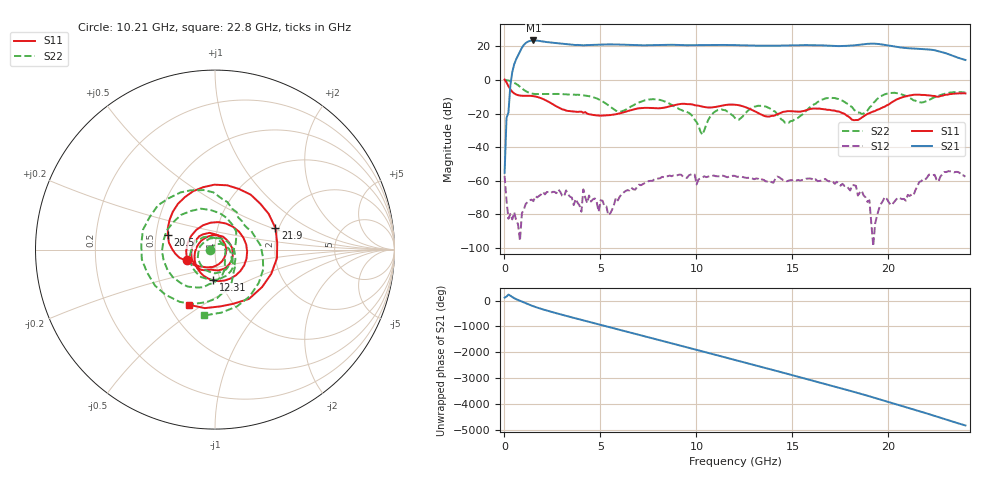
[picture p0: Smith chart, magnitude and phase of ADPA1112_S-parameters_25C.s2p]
! Analog Devices Inc.
! Device:  ADPA1112
! Description: 15 W, GaN Power Amplifier
! Frequency:  1 GHz to 22 GHz
! Package:
! Conditions:	Vdd = 28.0 V
!		Idd = 600 mA
!		Temp = +25 C
! The board loss has been subtracted from S21 Magnitude. Reference for all other parameters are at the connectors.
! Misc:JB
! Note: Analog Devices supplies this data as a sample of measured data for this product.
! Your particular data for this product may vary.
! Analog Devices reserves the right to change this data at anytime
! Freq(GHz)	S11a(dB)	S11p(deg)	S21a(dB)	S21p(deg)	S12a(dB)	S12p(deg)	S22a(dB)	S22p(deg)
# GHz S  dB  R 50
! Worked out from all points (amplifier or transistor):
!   241 points, 10 MHz to 24 GHz, reference 50 ohm
!   highest |S21| = 23.6 dB at 1.51 GHz (marker M1)
!   |S21| within 3 dB of that: 990.5 MHz to 12.74 GHz (11.75 GHz wide, 171 % of centre)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
!   unconditionally stable (mu >= 1): 108.8 MHz to end of sweep
!   at 4.009 GHz: K = 335.63, MAG = 21.4 dB, |S12| = -78.6 dB
!   at 12.01 GHz: K = 31.77, MAG = 21.0 dB, |S12| = -57.2 dB
!   at 24 GHz: K = 67.20, MAG = 13.5 dB, |S12| = -57.7 dB
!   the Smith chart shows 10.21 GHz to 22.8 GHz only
!   S11 on the Smith chart (normalised r, x): 10.21 GHz: 0.73, -0.08; 12.31 GHz: 0.92, -0.32; 20.5 GHz: 0.58, +0.10; 21.9 GHz: 1.92, +0.53; 22.8 GHz: 0.63, -0.44
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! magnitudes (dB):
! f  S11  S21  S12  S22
! 10 MHz  0.3  -55.4  -57.3  0.2
! 110 MHz  -1.4  -22.6  -72.0  -0.2
! 409.9 MHz  -7.1  4.8  -83.2  -1.1
! 1.51 GHz  -9.6  23.6  -72.3  -8.2
! 3.209 GHz  -18.2  21.4  -65.9  -8.5
! 4.009 GHz  -18.9  20.8  -78.6  -8.9
! 4.109 GHz  -19.6  20.7  -65.3  -9.2
! 5.409 GHz  -21.0  21.2  -80.6  -15.1
! 8.108 GHz  -16.8  20.9  -58.6  -11.9
! 10.21 GHz  -15.6  20.8  -58.7  -30.8
! 11.11 GHz  -15.8  20.9  -57.4  -17.9
! 12.01 GHz  -14.8  20.8  -57.2  -22.7
! 12.31 GHz  -15.3  20.8  -57.6  -22.7
! 14.81 GHz  -18.6  20.6  -60.0  -25.5
! 16.01 GHz  -17.1  20.8  -59.0  -15.4
! 18.61 GHz  -22.4  21.2  -66.1  -20.2
! 19.11 GHz  -19.3  21.7  -85.2  -15.4
! 20.1 GHz  -13.8  20.4  -74.6  -7.7
! 20.5 GHz  -11.2  19.6  -70.1  -7.9
! 21.9 GHz  -8.9  18.4  -59.5  -12.9
! 22.8 GHz  -9.4  16.6  -56.2  -8.6
! 24 GHz  -8.0  11.9  -57.7  -7.5
